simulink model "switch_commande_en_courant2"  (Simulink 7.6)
settings: Solver=ode15s  StartTime=0.0  StopTime=0.4  RelTol=1e-3
InitFcn:
  | C=100e-9;
  | R=10e3;
StopFcn:
  | close all, clc
  | load es.mat
  | plotyy(x(1,:),x(2,:),x(1,:),x(3,:))
  | grid
  | 
  | title('Switch commandé en courant')
  | xlabel('temps continu')
undefined symbols (not defined in the file or in its folder): sigbuilder_block
libraries: fl_lib x15, nesl_utility x5, elec_lib x1, simulink x1

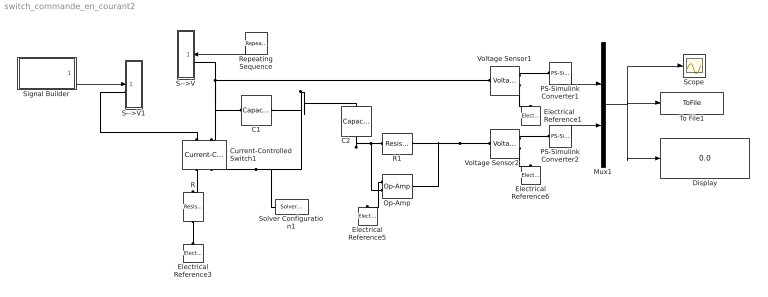
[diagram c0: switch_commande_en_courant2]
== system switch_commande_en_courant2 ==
  C1 : fl_lib/Electrical/Electrical Elements/Capacitor  DialogController=NetworkEngine.DynNeDlgSource  SystemSampleTime=-1  c=C F  v0=0 V  r=1e-6 Ohm  g=0 1/Ohm  i_Log=off  v_Log=off  vc_Log=off  LocalVarNames=|current|voltage|power  LocalVarDescs=|Capacitor current (A)|Voltage across capacitor (V)|Power (W)  LocalVarLogging=[0 0 0]
  C2 : fl_lib/Electrical/Electrical Elements/Capacitor  DialogController=NetworkEngine.DynNeDlgSource  SystemSampleTime=-1  c=C F  v0=0 V  r=1e-6 Ohm  g=0 1/Ohm  i_Log=off  v_Log=off  vc_Log=off  LocalVarNames=|current|voltage|power  LocalVarDescs=|Capacitor current (A)|Voltage across capacitor (V)|Power (W)  LocalVarLogging=[0 0 0]
  Current-Controlled Switch1 : elec_lib/Additional Components/SPICE-Compatible Components/Passive Devices/Current-Controlled Switch  DialogController=NetworkEngine.DynNeDlgSource  SystemSampleTime=-1  IT=0.5 mA  IH=0 A  RON=0.001 Ohm  ROFF=1e+12 Ohm  IC_state=-1  LocalVarLogging=[]
  Display : Display
  Electrical Reference{1,3,5..6} (4 alike) : fl_lib/Electrical/Electrical Elements/Electrical Reference  DialogController=NetworkEngine.DynNeDlgSource  SystemSampleTime=-1  i_Log=off  LocalVarNames=|i  LocalVarDescs=|i  LocalVarLogging=[]
  Mux1 : Mux  Inputs=2
  Op-Amp : fl_lib/Electrical/Electrical Elements/Op-Amp  DialogController=NetworkEngine.DynNeDlgSource  SystemSampleTime=-1  i1_Log=off  v1_Log=off  outI_Log=off  LocalVarNames=|i1|v1|outI  LocalVarDescs=|i1|v1|outI  LocalVarLogging=[]
  PS-Simulink Converter1 : nesl_utility/PS-Simulink Converter  DialogController=NetworkEngine.DynNeUtilDlgSource  SystemSampleTime=-1  PhysicalDomain=network_engine_domain  LeftPortType=input  RightPortType=output  SubClassName=ps_output  Unit=1  AffineConversion=off
  PS-Simulink Converter2 : nesl_utility/PS-Simulink Converter  DialogController=NetworkEngine.DynNeUtilDlgSource  SystemSampleTime=-1  PhysicalDomain=network_engine_domain  LeftPortType=input  RightPortType=output  SubClassName=ps_output  Unit=1  AffineConversion=off
  R : fl_lib/Electrical/Electrical Elements/Resistor  DialogController=NetworkEngine.DynNeDlgSource  SystemSampleTime=-1  R=1e3 Ohm  i_Log=off  v_Log=off  LocalVarNames=|current|voltage|power  LocalVarDescs=|Resistor current (A)|Voltage across resistor (V)|Power (W)  LocalVarLogging=[0 0 0]
  R1 : fl_lib/Electrical/Electrical Elements/Resistor  DialogController=NetworkEngine.DynNeDlgSource  SystemSampleTime=-1  R=R Ohm  i_Log=off  v_Log=off  LocalVarNames=|current|voltage|power  LocalVarDescs=|Resistor current (A)|Voltage across resistor (V)|Power (W)  LocalVarLogging=[0 0 0]
  Repeating Sequence : simulink/Sources/Repeating Sequence  SystemSampleTime=-1  rep_seq_t=[0 0.1 0.2 0.3 0.4]  rep_seq_y=[0 1 0 1 0]
  S-->V : Subsystem
  S-->V1 : Subsystem
  Scope : Scope
  Signal Builder : Subsystem  Tag=STV Subsys  LoadFcn=sigbuilder_block('load');  StartFcn=sigbuilder_block('start');  StopFcn=sigbuilder_block('stop');  ClipboardFcn=sigbuilder_block('clipboard');
  Solver Configuration1 : nesl_utility/Solver Configuration  DialogController=NetworkEngine.DynNeUtilDlgSource  SystemSampleTime=-1  PhysicalDomain=network_engine_domain  LeftPortType=input  RightPortType=generic  SubClassName=solver  Accelerate=off  Profile=off  ResidualTolerance=1e-9  MaxNonlinIter=12  MaxModeIter=2  DoFixedCost=off  UseLocalSampling=off  DoDC=off  LinearAlgebra=Sparse  LocalSolverSampleTime=.001  LocalSolverChoice=NE_BACKWARD_EULER_ADVANCER  UseLocalSolver=off
  To File1 : ToFile  Filename=es.mat  MatrixName=x
  Voltage Sensor1 : fl_lib/Electrical/Electrical Sensors/Voltage Sensor  DialogController=NetworkEngine.DynNeDlgSource  SystemSampleTime=-1  i1_Log=off  v1_Log=off  LocalVarNames=|i1|v1  LocalVarDescs=|i1|v1  LocalVarLogging=[]
  Voltage Sensor2 : fl_lib/Electrical/Electrical Sensors/Voltage Sensor  DialogController=NetworkEngine.DynNeDlgSource  SystemSampleTime=-1  i1_Log=off  v1_Log=off  LocalVarNames=|i1|v1  LocalVarDescs=|i1|v1  LocalVarLogging=[]
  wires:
  Repeating Sequence/1 -> S-->V/1(S)
  Signal Builder/1(Signal 2) -> S-->V1/1(S)
  Mux1/1 -> To File1/1, Scope/1, Display/1
  PS-Simulink Converter2/1 -> Mux1/2
  PS-Simulink Converter1/1 -> Mux1/1
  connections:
  R1/LConn1 -- Op-Amp/LConn2 -- C2/RConn1
  Op-Amp/LConn1 -- Electrical Reference5/LConn1
  R/RConn1 -- Electrical Reference3/LConn1
  Current-Controlled Switch1/RConn1 -- R/LConn1
  Current-Controlled Switch1/LConn1 -- S-->V1/LConn1
  Voltage Sensor2/RConn1 -- PS-Simulink Converter2/LConn1
  Voltage Sensor2/RConn2 -- Electrical Reference6/LConn1
  S-->V/LConn1 -- Voltage Sensor1/LConn1 -- Current-Controlled Switch1/LConn2 -- C1/LConn1
  Voltage Sensor1/RConn1 -- PS-Simulink Converter1/LConn1
  Voltage Sensor1/RConn2 -- Electrical Reference1/LConn1
  Current-Controlled Switch1/RConn2 -- C2/LConn1 -- C1/RConn1 -- Solver Configuration1/RConn1
  Voltage Sensor2/LConn1 -- R1/RConn1 -- Op-Amp/RConn1

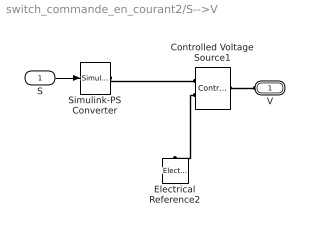
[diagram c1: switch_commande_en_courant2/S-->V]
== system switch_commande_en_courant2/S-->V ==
  S : Inport
  Controlled Voltage Source1 : fl_lib/Electrical/Electrical Sources/Controlled Voltage Source  DialogController=NetworkEngine.DynNeDlgSource  SystemSampleTime=-1  i_Log=off  v_Log=off  LocalVarNames=|current|voltage|power  LocalVarDescs=|Current (A)|Voltage (V)|Power (W)  LocalVarLogging=[0 0 0]
  Electrical Reference2 : fl_lib/Electrical/Electrical Elements/Electrical Reference  DialogController=NetworkEngine.DynNeDlgSource  SystemSampleTime=-1  i_Log=off  LocalVarNames=|i  LocalVarDescs=|i  LocalVarLogging=[]
  Simulink-PS Converter : nesl_utility/Simulink-PS Converter  DialogController=NetworkEngine.DynNeUtilDlgSource  SystemSampleTime=-1  PhysicalDomain=network_engine_domain  LeftPortType=input  RightPortType=output  SubClassName=ps_input  Unit=1  AffineConversion=off  InputFilterTimeConstant=.001  UdotUserProvided=0
  V : PMIOPort  Port=1  Side=Left
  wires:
  S/1 -> Simulink-PS Converter/1
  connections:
  Simulink-PS Converter/RConn1 -- Controlled Voltage Source1/RConn1
  Controlled Voltage Source1/RConn2 -- Electrical Reference2/LConn1
  V/RConn1 -- Controlled Voltage Source1/LConn1

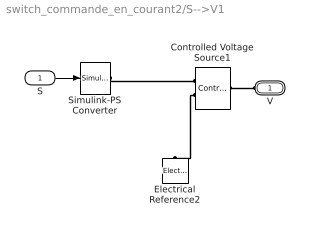
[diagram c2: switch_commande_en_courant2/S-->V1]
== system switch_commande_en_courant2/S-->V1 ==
  S : Inport
  Controlled Voltage Source1 : fl_lib/Electrical/Electrical Sources/Controlled Voltage Source  DialogController=NetworkEngine.DynNeDlgSource  SystemSampleTime=-1  i_Log=off  v_Log=off  LocalVarNames=|current|voltage|power  LocalVarDescs=|Current (A)|Voltage (V)|Power (W)  LocalVarLogging=[0 0 0]
  Electrical Reference2 : fl_lib/Electrical/Electrical Elements/Electrical Reference  DialogController=NetworkEngine.DynNeDlgSource  SystemSampleTime=-1  i_Log=off  LocalVarNames=|i  LocalVarDescs=|i  LocalVarLogging=[]
  Simulink-PS Converter : nesl_utility/Simulink-PS Converter  DialogController=NetworkEngine.DynNeUtilDlgSource  SystemSampleTime=-1  PhysicalDomain=network_engine_domain  LeftPortType=input  RightPortType=output  SubClassName=ps_input  Unit=1  AffineConversion=off  InputFilterTimeConstant=.001  UdotUserProvided=0
  V : PMIOPort  Port=1  Side=Left
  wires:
  S/1 -> Simulink-PS Converter/1
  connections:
  V/RConn1 -- Controlled Voltage Source1/LConn1
  Controlled Voltage Source1/RConn2 -- Electrical Reference2/LConn1
  Simulink-PS Converter/RConn1 -- Controlled Voltage Source1/RConn1

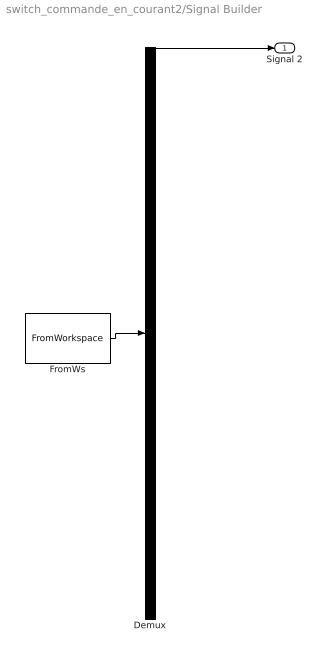
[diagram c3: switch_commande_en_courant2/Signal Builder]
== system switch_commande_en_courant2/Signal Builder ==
  Demux : Demux  Tag=STV Demux  Outputs=1
  FromWs : FromWorkspace  Tag=STV FromWs  VariableName=tuvar  SampleTime=0  SigBuilderData=DataTag0  VnvData=DataTag1
  Signal 2 : Outport  Tag=STV Outport
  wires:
  FromWs/1 -> Demux/1
  Demux/1 -> Signal 2/1
